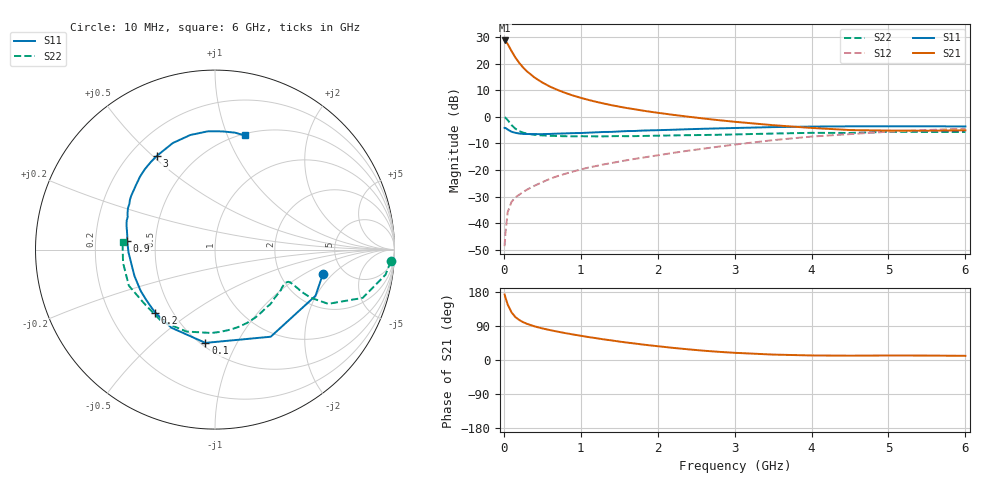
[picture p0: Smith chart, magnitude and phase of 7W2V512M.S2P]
! Infineon Technologies  Discrete & RF Semiconductors
! BFS17W
! Si NPN RF Bipolar Junction Transistor in SOT323
! VCE = 2.5 V  IC = 12 mA
! Common Emitter S-Parameters:  August  1999
# GHz  S  MA  R  50
!  f  S11  S21  S12  S22
! GHz  MAG  ANG  MAG  ANG  MAG  ANG  MAG  ANG
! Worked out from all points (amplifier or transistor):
!   36 points, 10 MHz to 6 GHz, reference 50 ohm
!   highest |S21| = 28.7 dB at 10 MHz (marker M1)
!   |S21| within 3 dB of that: start of sweep to 81.45 MHz
!   unconditionally stable (mu >= 1): 351.7 MHz to 2.643 GHz; 4.281 GHz to end of sweep
!   at 250 MHz: K = 0.86, MSG = 23.4 dB, |S12| = -28.3 dB
!   at 1.4 GHz: K = 1.22, MAG = 8.0 dB, |S12| = -17.4 dB
!   at 6 GHz: K = 1.08, MAG = -2.0 dB, |S12| = -4.5 dB
!   S11 on the Smith chart (normalised r, x): 10 MHz: 3.52, -1.52; 100 MHz: 0.53, -0.75; 200 MHz: 0.40, -0.37; 900 MHz: 0.34, +0.04; 3 GHz: 0.31, +0.51; 6 GHz: 0.51, +1.15
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0.01  0.6169 -12.5  27.12 173.0  0.0037 80.3  0.982 -3.8
0.02  0.6163 -24.7  26.55 165.4  0.0063 81.1  0.9602 -8.4
0.05  0.5762 -57.4  23.25 146.4  0.0161 68.4  0.8658 -18.1
0.1  0.5225 -95.9  17.15 125.7  0.0252 54.8  0.6994 -25.6
0.15  0.4985 -119.2  12.96 113.3  0.0306 53.3  0.5958 -26.7
0.2  0.4843 -133.6  10.27 105.6  0.0343 54.0  0.5381 -26.0
0.25  0.4749 -143.7  8.427 99.9  0.0385 54.5  0.5024 -24.9
0.3  0.4736 -151.0  7.135 95.5  0.0426 56.6  0.4824 -24.3
0.4  0.4722 -161.6  5.448 88.7  0.0507 59.5  0.4565 -23.5
0.5  0.4718 -168.5  4.399 83.4  0.059 61.9  0.4464 -23.7
0.6  0.4757 -173.8  3.679 78.9  0.0683 63.2  0.4386 -24.5
0.7  0.4822 -178.1  3.181 74.8  0.0768 64.7  0.434 -25.9
0.9  0.4926 174.3  2.5 67.4  0.0935 65.6  0.4288 -29.6
1.1  0.5023 167.7  2.07 60.6  0.1109 66.3  0.4286 -34.3
1.3  0.5176 162.0  1.77 54.4  0.1273 66.6  0.428 -39.6
1.6  0.5376 154.3  1.456 46.0  0.1525 67.0  0.4311 -47.9
2.2  0.5695 140.3  1.086 32.0  0.2093 67.0  0.4459 -66.5
3  0.6142 122.0  0.804 19.0  0.2997 63.1  0.465 -92.3
3.5  0.6387 111.6  0.694 14.3  0.3633 58.5  0.4834 -109.2
4.5  0.6603 93.4  0.562 11.4  0.4719 45.9  0.4961 -143.2
5.5  0.6611 80.4  0.546 11.7  0.5622 33.5  0.5176 -171.9
6  0.6574 75.5  0.557 11.0  0.598 27.6  0.5166 175.6
